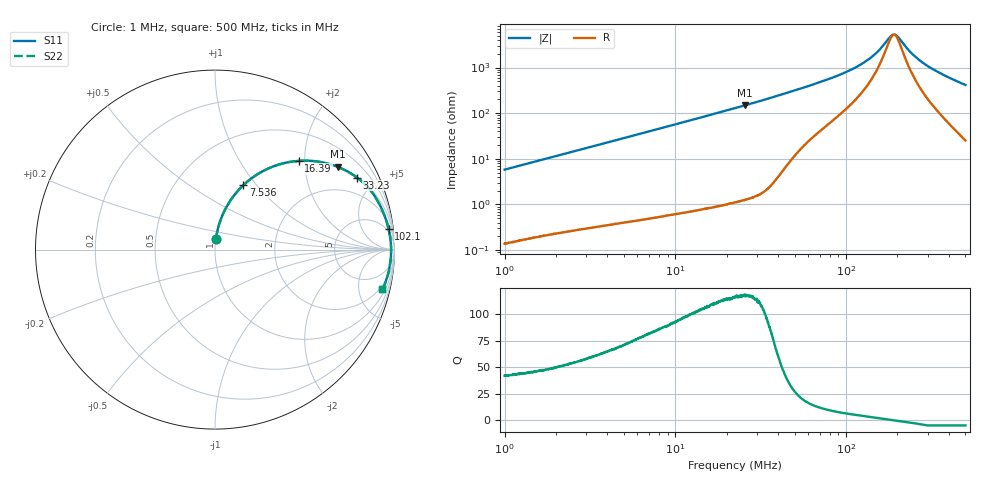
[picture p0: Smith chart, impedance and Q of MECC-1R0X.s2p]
!s-Parameter Generated by FASTRON Sdn. Bhd.
!FASTRON P/N : MECC-1R0X
!Keysight Technologies,E4991B,MY54100416,A.01.15
!Date: Mon Mar 16 14:41:15 2026
!Version  : Rev00 Mon Mar 16 14:41:15 2026
!Data & Calibration Information:
!PortZ  Port1:50+j0  Port2:50+j0
!When reading, reference impedance value at option line is always used.
!Remarks : This data is being provided solely for informational purposes.
!Freq	S11	S21	S12	S22
# Hz S dB R 50
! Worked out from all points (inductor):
!   1601 points, 1 MHz to 500 MHz, reference 50 ohm
!   read as one part in series: L = 918 nH near 1.032 MHz
!   highest Q = 118 at 25.42 MHz (marker M1), where L = 922 nH
!   self-resonance near 191 MHz
!   S11 on the Smith chart (normalised r, x): 1 MHz: 1.00, +0.12; 7.536 MHz: 1.01, +0.86; 16.39 MHz: 1.02, +1.87; 33.23 MHz: 1.04, +3.93; 102.1 MHz: 4, +16; 500 MHz: 1.50, -8.28
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1000000  -24.77 85.3  -0.03 -3.3  -0.03 -3.3  -24.77 85.3
2820919  -15.99 79.9  -0.14 -9.1  -0.14 -9.1  -15.99 79.9
4859040  -11.52 73.8  -0.35 -15.4  -0.35 -15.4  -11.52 73.8
7536423  -8.14 66.2  -0.77 -23.1  -0.77 -23.1  -8.14 66.2
7957584  -7.74 65.1  -0.85 -24.2  -0.85 -24.2  -7.74 65.1
1.115675e7  -5.46 57.2  -1.51 -32.2  -1.51 -32.2  -5.46 57.2
1.63884e7  -3.35 46.6  -2.77 -42.8  -2.77 -42.8  -3.35 46.6
2.236068e7  -2.09 37.7  -4.28 -51.9  -4.28 -51.9  -2.09 37.7
2.541858e7  -1.68 34.0  -5.04 -55.5  -5.04 -55.5  -1.68 34.0
3.323107e7  -1.03 26.8  -6.91 -62.6  -6.91 -62.6  -1.03 26.8
4.481592e7  -0.60 19.7  -9.45 -68.9  -9.45 -68.9  -0.60 19.7
6.307767e7  -0.38 13.3  -12.76 -72.8  -12.76 -72.8  -0.38 13.3
1.021047e8  -0.23 6.7  -18.54 -74.0  -18.54 -74.0  -0.23 6.7
1.404003e8  -0.18 3.2  -24.60 -67.9  -24.60 -67.9  -0.18 3.2
1.5714e8  -0.17 2.0  -27.95 -59.7  -27.95 -59.7  -0.17 2.0
1.77937e8  -0.16 0.7  -32.90 -33.8  -32.90 -33.8  -0.16 0.7
1.871524e8  -0.16 0.2  -34.43 -10.9  -34.43 -10.9  -0.16 0.2
1.96082e8  -0.16 -0.3  -34.35 14.6  -34.35 14.6  -0.16 -0.3
2.390382e8  -0.17 -2.4  -26.76 64.3  -26.76 64.3  -0.17 -2.4
2.835887e8  -0.18 -4.4  -22.10 72.8  -22.10 72.8  -0.18 -4.4
3.6362e8  -0.22 -7.7  -17.35 75.3  -17.35 75.3  -0.22 -7.7
5e8  -0.36 -13.4  -12.72 73.2  -12.72 73.2  -0.36 -13.4
